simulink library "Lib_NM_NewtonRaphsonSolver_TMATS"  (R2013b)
settings: Solver=ode45  StartTime=0.0  StopTime=10.0  RelTol=1e-3
undefined symbols (not defined in the file or in its folder): NR_dx_Lim_M, NR_IC_M

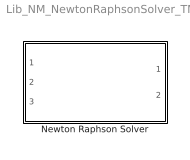
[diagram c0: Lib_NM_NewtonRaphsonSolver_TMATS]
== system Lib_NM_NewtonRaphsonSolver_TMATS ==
  Newton Raphson Solver : Subsystem  TreatAsAtomicUnit=on

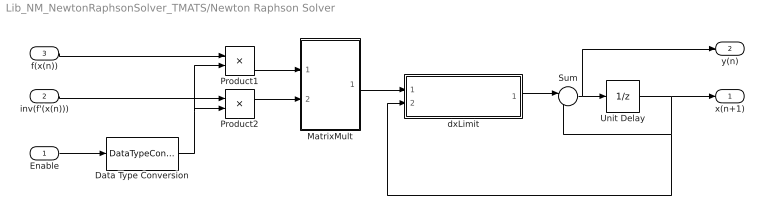
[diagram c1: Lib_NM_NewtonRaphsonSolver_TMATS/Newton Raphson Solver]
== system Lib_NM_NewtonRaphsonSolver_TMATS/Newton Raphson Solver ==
  Enable : Inport
  inv(f'(x(n))) : Inport  Port=2
  f(x(n)) : Inport  Port=3
  Data Type Conversion : DataTypeConversion
  MatrixMult : Subsystem
  Product1 : Product
  Product2 : Product
  Sum : Sum  Inputs=|-+
  Unit Delay : UnitDelay  InitialCondition=NR_IC_M  SampleTime=-1
  dxLimit : Subsystem
  x(n+1) : Outport
  y(n) : Outport  Port=2
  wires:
  inv(f'(x(n)))/1 -> Product2/1
  f(x(n))/1 -> Product1/1
  MatrixMult/1(DTS) -> dxLimit/1(dx)
  dxLimit/1(dx_limited) -> Sum/1
  Sum/1 -> y(n)/1, Unit Delay/1
  Unit Delay/1 -> Sum/2, dxLimit/2(dx1), x(n+1)/1
  Product1/1 -> MatrixMult/1(f(x(n)))
  Product2/1 -> MatrixMult/2(inv(f'(x(n))))
  Enable/1 -> Data Type Conversion/1
  Data Type Conversion/1 -> Product1/2, Product2/2

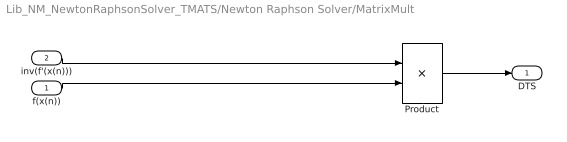
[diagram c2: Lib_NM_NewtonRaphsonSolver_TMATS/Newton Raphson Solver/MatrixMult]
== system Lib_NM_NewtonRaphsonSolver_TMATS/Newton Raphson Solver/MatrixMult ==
  f(x(n)) : Inport
  inv(f'(x(n))) : Inport  Port=2
  Product : Product  Multiplication=Matrix(*)
  DTS : Outport
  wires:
  Product/1 -> DTS/1
  f(x(n))/1 -> Product/2
  inv(f'(x(n)))/1 -> Product/1

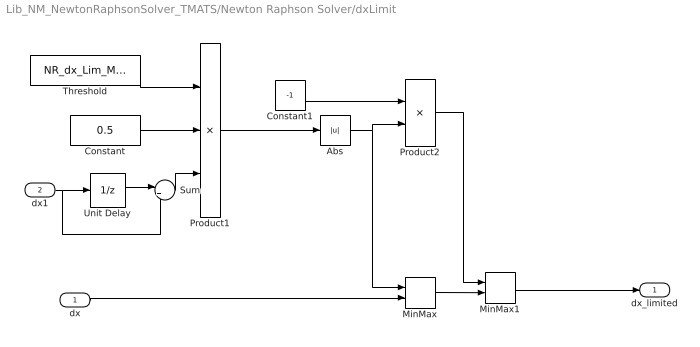
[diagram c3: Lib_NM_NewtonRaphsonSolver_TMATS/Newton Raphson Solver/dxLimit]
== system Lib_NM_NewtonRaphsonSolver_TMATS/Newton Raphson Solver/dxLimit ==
  dx : Inport
  dx1 : Inport  Port=2
  Abs : Abs
  Constant : Constant  Value=0.5
  Constant1 : Constant  Value=-1
  MinMax : MinMax  Inputs=2
  MinMax1 : MinMax  Function=max  Inputs=2
  Product1 : Product  Inputs=3
  Product2 : Product
  Sum : Sum  Inputs=|++
  Threshold : Constant  Value=NR_dx_Lim_M/100
  Unit Delay : UnitDelay  InitialCondition=NR_IC_M  SampleTime=-1
  dx_limited : Outport
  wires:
  MinMax1/1 -> dx_limited/1
  Constant1/1 -> Product2/1
  Product2/1 -> MinMax1/1
  MinMax/1 -> MinMax1/2
  dx/1 -> MinMax/2
  Abs/1 -> Product2/2, MinMax/1
  Product1/1 -> Abs/1
  Threshold/1 -> Product1/1
  dx1/1 -> Sum/2, Unit Delay/1
  Constant/1 -> Product1/2
  Unit Delay/1 -> Sum/1
  Sum/1 -> Product1/3
